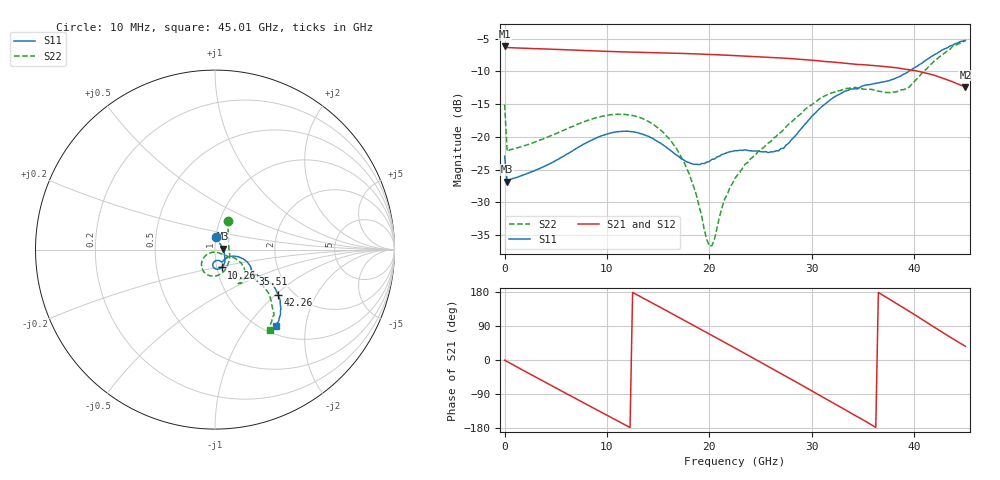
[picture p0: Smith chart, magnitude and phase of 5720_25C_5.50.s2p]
! Device:  ADRF5720
! Description: 0.5dB LSB GaAs MMIC 6-bit Digital Attenuator
! Frequency:  0.000009 -  40 GHz
! Ports:
!	RF1	= Port 1
!	RF2	= Port 2
! Vdd:  3.3 Volt
! Vss:  -3.3 Volt
! Control:  0/3.3 Volt
! State:  5.50 dB attenuation
! Data:  The device was measured using G-S-G Probes on a matrix board.
!  Data was collected using an calibrated 4 port network analyzer.
!  The reference plane for this measurement is at the launchers.
! Note:  Analog Devices supplies this data as a sample of measured data
!  for this product.  Your particular data for this product may vary.
!  Data was taken at 25 degrees C.
!  Analog Devices reserves the right to change this data at anytime.
# GHZ S DB R 45.0
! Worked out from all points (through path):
!   181 points, 10 MHz to 45.01 GHz, reference 45 ohm
!   highest |S21| = -6.18 dB at 10 MHz (marker M1); lowest = -12.4 dB at 45.01 GHz (marker M2)
!   group delay of S21, straight-line fit = 41.8 ps
!   lowest |S11| = -26.8 dB at 260 MHz (marker M3), VSWR 1.10, Z = 49.3 + j0.543 ohm
!   |S11| at or under -10 dB: start of sweep to 39.48 GHz
!   |S22| runs from -36.7 to -5.3 dB; largest |S21 - S12| = 0.00054
!   S11 on the Smith chart (normalised r, x): 10 MHz: 1.00, +0.14; 10.26 GHz: 1.05, -0.21; 35.51 GHz: 1.46, -0.42; 42.26 GHz: 1.68, -1.05; 45.01 GHz: 1.15, -1.38
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0.01  -22.94 87.6  -6.18 -0.6  -6.18 -0.6  -15.06 66.1
0.26  -26.82 6.9  -6.37 -4.1  -6.37 -4.1  -22.24 2.6
2.01  -25.73 -13.4  -6.48 -30.0  -6.48 -30.0  -21.32 -17.7
4.26  -24.23 -30.5  -6.61 -62.8  -6.61 -62.8  -20.01 -39.0
7.76  -21.09 -51.9  -6.82 -113.4  -6.82 -113.4  -17.69 -67.7
10.26  -19.47 -69.7  -6.97 -149.4  -6.97 -149.4  -16.65 -88.6
12.76  -19.30 -87.2  -7.09 174.6  -7.09 174.6  -16.84 -110.5
15.26  -20.98 -98.2  -7.18 138.3  -7.18 138.3  -18.99 -132.2
18.01  -23.93 -88.7  -7.31 98.1  -7.31 98.1  -25.58 -148.8
20.01  -23.76 -69.8  -7.42 68.5  -7.42 68.5  -36.69 -99.2
20.51  -23.38 -67.1  -7.46 61.1  -7.46 61.1  -35.62 -58.6
21.51  -22.56 -63.5  -7.53 46.4  -7.53 46.4  -29.47 -37.7
22.76  -22.11 -61.4  -7.61 27.8  -7.61 27.8  -25.82 -30.3
26.26  -22.30 -42.2  -7.89 -24.5  -7.89 -24.4  -20.19 -24.4
28.26  -20.07 -22.1  -8.09 -54.7  -8.09 -54.7  -17.40 -24.8
30.26  -16.50 -17.2  -8.34 -85.3  -8.34 -85.2  -14.77 -30.5
32.51  -13.65 -23.5  -8.65 -119.6  -8.65 -119.5  -12.98 -41.7
35.51  -12.06 -32.4  -9.04 -165.9  -9.05 -165.9  -12.72 -54.1
37.76  -11.29 -32.1  -9.37 157.9  -9.37 158.0  -13.30 -49.8
40.26  -9.27 -30.6  -9.94 116.0  -9.94 116.1  -11.18 -36.1
42.26  -7.24 -35.7  -10.75 81.5  -10.75 81.6  -8.09 -39.8
45.01  -5.29 -51.1  -12.39 36.2  -12.39 36.2  -5.35 -55.7
